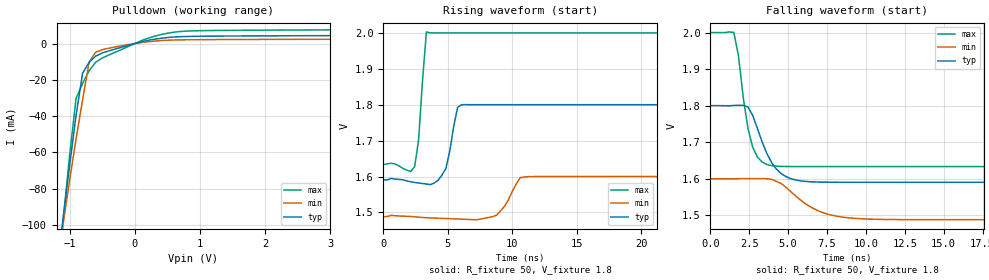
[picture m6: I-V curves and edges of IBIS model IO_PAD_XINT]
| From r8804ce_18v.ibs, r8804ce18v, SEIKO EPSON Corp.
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[Model]   IO_PAD_XINT
Model_type Open_drain
Enable Active-High
Polarity Non-Inverting
Vref=2.0
Vmeas=0.90
Rref=5000
C_comp   2.5p   2.0p   3.0p
[Temperature Range] 25   105   -40
[Voltage Range]   1.8   1.6   2.0
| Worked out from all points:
|   slope of the pulldown table from 0 to 0.27 V, typ, clamps not added: 124 ohm
|   falling waveform, R_fixture 50, V_fixture 1.8: 20-80 % time 1.29ns typ, 2.21ns min, 764ps max; typ from 1.8 V to 1.59 V
|   rising waveform, R_fixture 50, V_fixture 1.8: 20-80 % time 652ps typ, 1.05ns min, 428ps max; typ from 1.59 V to 1.8 V
[Pulldown]
-1.8V     -315.9mA   -273.2mA   -373.7mA
-1.2V     -127.2mA   -124.2mA   -134.4mA
-1.1V     -96.62mA   -99.76mA   -98.16mA
-1V       -67.5mA    -75.64mA   -61.98mA
-900mV    -39.61mA   -52.59mA   -30.27mA
-800mV    -16.38mA   -31.06mA   -22mA
-700mV    -10.39mA   -10.33mA   -15.04mA
-600mV    -6.971mA   -4.809mA   -10.32mA
-400mV    -4.076mA   -2.558mA   -6.371mA
100mV     923.1uA    534.4uA    1.541mA
600mV     3.612mA    1.975mA    6.261mA
3.6V      4.437mA    2.42mA     7.642mA
[Falling Waveform]
R_fixture=50
V_fixture=1.8
V_fixture_min=1.6
V_fixture_max=2.0
0s        1.8V       1.6V       2V
1.515ns   1.801V     1.6V       2V
1.818ns   1.801V     1.6V       1.935V
2.424ns   1.796V     1.6V       1.737V
3.03ns    1.738V     1.6V       1.659V
3.636ns   1.669V     1.6V       1.639V
5.152ns   1.6V       1.565V     1.633V
6.97ns    1.591V     1.512V     1.633V
9.091ns   1.59V      1.492V     1.633V
30ns      1.59V      1.488V     1.633V
[Rising Waveform]
R_fixture=50
V_fixture=1.8
V_fixture_min=1.6
V_fixture_max=2.0
0s        1.59V      1.488V     1.633V
2.424ns   1.583V     1.488V     1.628V
2.727ns   1.582V     1.487V     1.701V
3.333ns   1.579V     1.485V     2.003V
4.848ns   1.623V     1.483V     2V
5.758ns   1.793V     1.482V     2V
6.061ns   1.8V       1.481V     2V
8.788ns   1.8V       1.492V     2V
10.91ns   1.8V       1.599V     2V
30ns      1.8V       1.6V       2V
[Ramp]
R_load=50
dV/dt_r   1.258E-1/6.197E-10   6.722E-2/1.044E-9   2.200E-1/3.832E-10
dV/dt_f   1.258E-1/1.274E-9   6.722E-2/2.199E-9   2.200E-1/7.444E-10
|[End   IO_PAD_XINT
